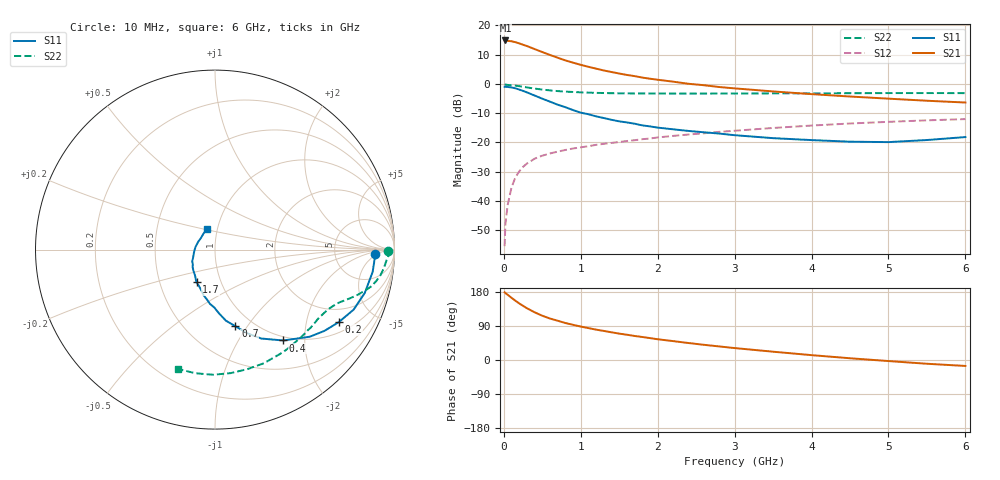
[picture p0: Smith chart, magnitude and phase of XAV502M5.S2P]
! SIEMENS Discrete & RF Semiconductors
! BFY180
! Si NPN RF Bipolar Junction Transistor in MICRO-X
! VCE = 0.5 V  IC = 2.5 mA
! Common Emitter S-Parameters:  May  1997
# GHz  S  MA  R  50
!  f  S11  S21  S12  S22
! GHz  MAG  ANG  MAG  ANG  MAG  ANG  MAG  ANG
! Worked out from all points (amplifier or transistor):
!   36 points, 10 MHz to 6 GHz, reference 50 ohm
!   highest |S21| = 14.8 dB at 20 MHz (marker M1)
!   |S21| within 3 dB of that: start of sweep to 405.6 MHz
!   unconditionally stable (mu >= 1): 620.9 MHz to end of sweep
!   at 250 MHz: K = 0.46, MSG = 20.8 dB, |S12| = -28.3 dB
!   at 1.4 GHz: K = 1.67, MAG = 7.3 dB, |S12| = -20.1 dB
!   at 6 GHz: K = 2.08, MAG = -3.1 dB, |S12| = -12.0 dB
!   S11 on the Smith chart (normalised r, x): 10 MHz: 17, -4; 200 MHz: 1.39, -3.12; 400 MHz: 0.93, -1.58; 700 MHz: 0.83, -0.88; 1.7 GHz: 0.77, -0.29; 6 GHz: 0.89, +0.21
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0.01  0.8919 -1.6  5.426 178.6  0.0017 87.5  0.9619 -0.5
0.02  0.891 -3.3  5.515 176.7  0.004 91.9  0.9742 -1.2
0.05  0.8872 -8.0  5.416 172.1  0.0086 83.0  0.96 -3.0
0.1  0.8689 -16.1  5.345 164.1  0.0172 80.0  0.9473 -6.1
0.15  0.8418 -23.4  5.15 156.5  0.0253 74.1  0.9335 -8.7
0.2  0.7996 -30.3  4.919 149.3  0.0321 69.8  0.9147 -11.1
0.3  0.7172 -42.6  4.431 136.6  0.0437 61.9  0.8705 -15.0
0.4  0.6333 -53.1  3.93 125.9  0.0529 57.5  0.8323 -17.7
0.5  0.5586 -62.5  3.495 116.8  0.0596 53.1  0.8 -19.8
0.6  0.4979 -69.1  3.118 109.4  0.065 50.2  0.7742 -21.5
0.7  0.4419 -75.1  2.798 103.6  0.0698 48.4  0.7541 -22.9
0.8  0.4003 -81.3  2.517 97.6  0.0746 47.1  0.7388 -24.3
0.9  0.3569 -86.3  2.303 92.8  0.079 46.0  0.7279 -25.7
1.1  0.3036 -95.3  1.955 84.2  0.0864 44.7  0.7099 -28.5
1.4  0.244 -107.5  1.595 73.1  0.0983 43.4  0.6934 -33.0
1.7  0.2093 -119.4  1.358 63.4  0.1094 42.3  0.6871 -37.5
2.2  0.1679 -135.9  1.092 49.9  0.1296 39.7  0.6836 -45.8
2.8  0.142 -153.6  0.885 35.8  0.1519 36.1  0.6851 -55.4
3.5  0.1186 -172.0  0.744 21.9  0.177 31.2  0.6892 -66.7
4.5  0.1032 154.8  0.609 4.6  0.2109 22.4  0.6937 -82.7
5.5  0.1102 125.3  0.516 -9.9  0.2388 13.4  0.6975 -99.1
6  0.1238 110.4  0.481 -15.7  0.2508 8.7  0.696 -107.1
